FUNCTION_BLOCK FB 1
TITLE =
AUTHOR : gersch
FAMILY : 'cpu/ap'
NAME : gfpv
VERSION : 7.0

BEGIN
NETWORK
TITLE =
//***                                                                         ***
//***                    schunk antriebssystem: fb20 test funktion            ***
//***                                                                         ***


NETWORK
TITLE =schunk antrieb: datenaustausch sps/modul PEB
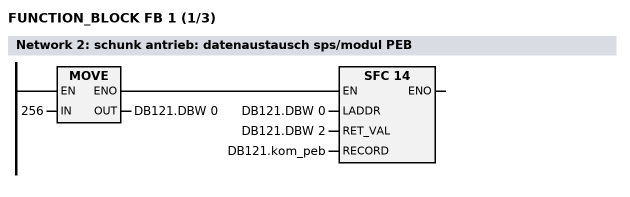
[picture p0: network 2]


      L     256;
      T     DB121.DBW    0;
      CALL SFC   14 (
           LADDR                    := DB121.DBW    0,
           RET_VAL                  := DB121.DBW    2,
           RECORD                   := DB121.kom_peb);

NETWORK
TITLE =schunk antriebs ansteuerung
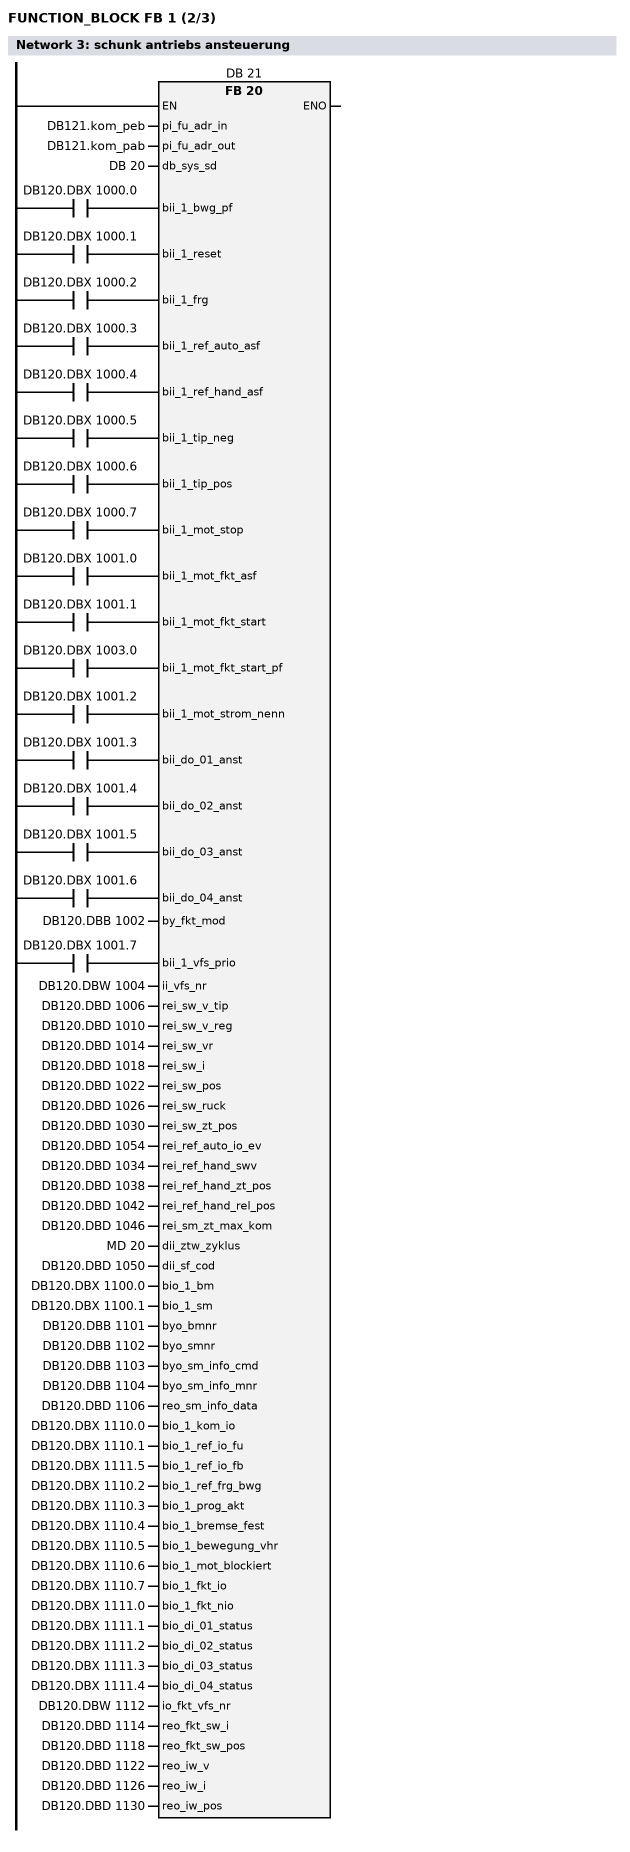
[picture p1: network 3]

      U     DB120.DBX 1000.0;
      =     L      0.0;
      BLD   103;
      U     DB120.DBX 1000.1;
      =     L      0.1;
      BLD   103;
      U     DB120.DBX 1000.2;
      =     L      0.2;
      BLD   103;
      U     DB120.DBX 1000.3;
      =     L      0.3;
      BLD   103;
      U     DB120.DBX 1000.4;
      =     L      0.4;
      BLD   103;
      U     DB120.DBX 1000.5;
      =     L      0.5;
      BLD   103;
      U     DB120.DBX 1000.6;
      =     L      0.6;
      BLD   103;
      U     DB120.DBX 1000.7;
      =     L      0.7;
      BLD   103;
      U     DB120.DBX 1001.0;
      =     L      1.0;
      BLD   103;
      U     DB120.DBX 1001.1;
      =     L      1.1;
      BLD   103;
      U     DB120.DBX 1003.0;
      =     L      1.2;
      BLD   103;
      U     DB120.DBX 1001.2;
      =     L      1.3;
      BLD   103;
      U     DB120.DBX 1001.3;
      =     L      1.4;
      BLD   103;
      U     DB120.DBX 1001.4;
      =     L      1.5;
      BLD   103;
      U     DB120.DBX 1001.5;
      =     L      1.6;
      BLD   103;
      U     DB120.DBX 1001.6;
      =     L      1.7;
      BLD   103;
      U     DB120.DBX 1001.7;
      =     L      2.0;
      BLD   103;
      CALL FB    20 , DB    21 (
           pi_fu_adr_in             := DB121.kom_peb,
           pi_fu_adr_out            := DB121.kom_pab,
           db_sys_sd                := DB    20,
           bii_1_bwg_pf             := L      0.0,
           bii_1_reset              := L      0.1,
           bii_1_frg                := L      0.2,
           bii_1_ref_auto_asf       := L      0.3,
           bii_1_ref_hand_asf       := L      0.4,
           bii_1_tip_neg            := L      0.5,
           bii_1_tip_pos            := L      0.6,
           bii_1_mot_stop           := L      0.7,
           bii_1_mot_fkt_asf        := L      1.0,
           bii_1_mot_fkt_start      := L      1.1,
           bii_1_mot_fkt_start_pf   := L      1.2,
           bii_1_mot_strom_nenn     := L      1.3,
           bii_do_01_anst           := L      1.4,
           bii_do_02_anst           := L      1.5,
           bii_do_03_anst           := L      1.6,
           bii_do_04_anst           := L      1.7,
           by_fkt_mod               := DB120.DBB 1002,
           bii_1_vfs_prio           := L      2.0,
           ii_vfs_nr                := DB120.DBW 1004,
           rei_sw_v_tip             := DB120.DBD 1006,
           rei_sw_v_reg             := DB120.DBD 1010,
           rei_sw_vr                := DB120.DBD 1014,
           rei_sw_i                 := DB120.DBD 1018,
           rei_sw_pos               := DB120.DBD 1022,
           rei_sw_ruck              := DB120.DBD 1026,
           rei_sw_zt_pos            := DB120.DBD 1030,
           rei_ref_auto_io_ev       := DB120.DBD 1054,
           rei_ref_hand_swv         := DB120.DBD 1034,
           rei_ref_hand_zt_pos      := DB120.DBD 1038,
           rei_ref_hand_rel_pos     := DB120.DBD 1042,
           rei_sm_zt_max_kom        := DB120.DBD 1046,
           dii_ztw_zyklus           := MD    20,
           dii_sf_cod               := DB120.DBD 1050,
           bio_1_bm                 := DB120.DBX 1100.0,
           bio_1_sm                 := DB120.DBX 1100.1,
           byo_bmnr                 := DB120.DBB 1101,
           byo_smnr                 := DB120.DBB 1102,
           byo_sm_info_cmd          := DB120.DBB 1103,
           byo_sm_info_mnr          := DB120.DBB 1104,
           reo_sm_info_data         := DB120.DBD 1106,
           bio_1_kom_io             := DB120.DBX 1110.0,
           bio_1_ref_io_fu          := DB120.DBX 1110.1,
           bio_1_ref_io_fb          := DB120.DBX 1111.5,
           bio_1_ref_frg_bwg        := DB120.DBX 1110.2,
           bio_1_prog_akt           := DB120.DBX 1110.3,
           bio_1_bremse_fest        := DB120.DBX 1110.4,
           bio_1_bewegung_vhr       := DB120.DBX 1110.5,
           bio_1_mot_blockiert      := DB120.DBX 1110.6,
           bio_1_fkt_io             := DB120.DBX 1110.7,
           bio_1_fkt_nio            := DB120.DBX 1111.0,
           bio_di_01_status         := DB120.DBX 1111.1,
           bio_di_02_status         := DB120.DBX 1111.2,
           bio_di_03_status         := DB120.DBX 1111.3,
           bio_di_04_status         := DB120.DBX 1111.4,
           io_fkt_vfs_nr            := DB120.DBW 1112,
           reo_fkt_sw_i             := DB120.DBD 1114,
           reo_fkt_sw_pos           := DB120.DBD 1118,
           reo_iw_v                 := DB120.DBD 1122,
           reo_iw_i                 := DB120.DBD 1126,
           reo_iw_pos               := DB120.DBD 1130);
      NOP   0;
NETWORK
TITLE =schunk antrieb: datenaustausch sps/modul PAB
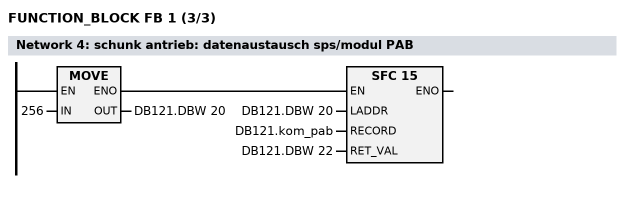
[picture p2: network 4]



      L     256;
      T     DB121.DBW   20;
      CALL SFC   15 (
           LADDR                    := DB121.DBW   20,
           RECORD                   := DB121.kom_pab,
           RET_VAL                  := DB121.DBW   22);

END_FUNCTION_BLOCK

